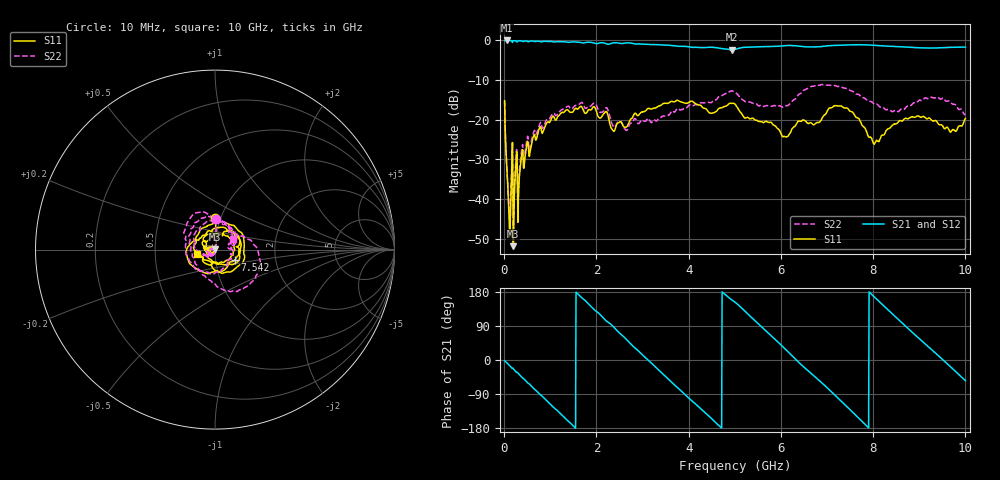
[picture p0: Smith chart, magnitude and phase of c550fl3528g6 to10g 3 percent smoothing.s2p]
!Agilent Technologies,N5234A,MY52241123,A.10.00.00
!Agilent N5234A: A.10.00.00
!Date: Wednesday, August 14, 2019 08:09:08
!Correction: S11(Full 2 Port(1,2))
!S21(Full 2 Port(1,2))
!S12(Full 2 Port(1,2))
!S22(Full 2 Port(1,2))
!S2P File: Measurements: S11, S21, S12, S22:
# Hz S  dB  R 50
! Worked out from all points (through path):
!   1001 points, 10 MHz to 10 GHz, reference 50 ohm
!   highest |S21| = -0.03 dB at 59.95 MHz (marker M1); lowest = -2.4 dB at 4.935 GHz (marker M2)
!   group delay of S21, straight-line fit = 314 ps
!   lowest |S11| = -51.9 dB at 199.8 MHz (marker M3), VSWR 1.01, Z = 50.1 + j0.22 ohm
!   |S11| at or under -10 dB: start of sweep to end of sweep
!   |S22| runs from -51.0 to -11.1 dB; largest |S21 - S12| = 0.0031
!   S11 on the Smith chart (normalised r, x): 10 MHz: 0.94, +0.34; 7.542 GHz: 1.24, -0.14; 10 GHz: 0.82, -0.04
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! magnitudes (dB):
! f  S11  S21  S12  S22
! 10 MHz  -15.2  -0.1  -0.1  -15.3
! 59.95 MHz  -32.5  0.0  0.0  -32.7
! 109.9 MHz  -45.6  0.0  -0.1  -43.5
! 159.8 MHz  -34.8  -0.1  -0.1  -33.8
! 199.8 MHz  -51.9  -0.1  -0.1  -51.0
! 759.2 MHz  -22.3  -0.2  -0.2  -21.4
! 1.678 GHz  -16.7  -0.6  -0.6  -15.7
! 2.208 GHz  -17.9  -0.8  -0.8  -17.0
! 2.368 GHz  -22.9  -0.6  -0.6  -21.8
! 3.347 GHz  -16.6  -1.1  -1.1  -19.7
! 4.505 GHz  -18.4  -1.7  -1.8  -15.5
! 4.935 GHz  -15.9  -2.4  -2.4  -12.7
! 5.005 GHz  -16.1  -2.3  -2.3  -13.1
! 6.074 GHz  -24.2  -1.3  -1.3  -16.6
! 6.673 GHz  -21.0  -1.7  -1.7  -11.6
! 7.173 GHz  -16.4  -1.3  -1.3  -11.4
! 7.542 GHz  -18.0  -1.1  -1.1  -12.8
! 8.022 GHz  -26.2  -1.2  -1.3  -16.1
! 8.342 GHz  -22.3  -1.5  -1.5  -17.4
! 9.371 GHz  -20.3  -1.9  -1.9  -14.4
! 9.71 GHz  -22.7  -1.7  -1.8  -16.0
! 10 GHz  -19.7  -1.7  -1.7  -18.7
